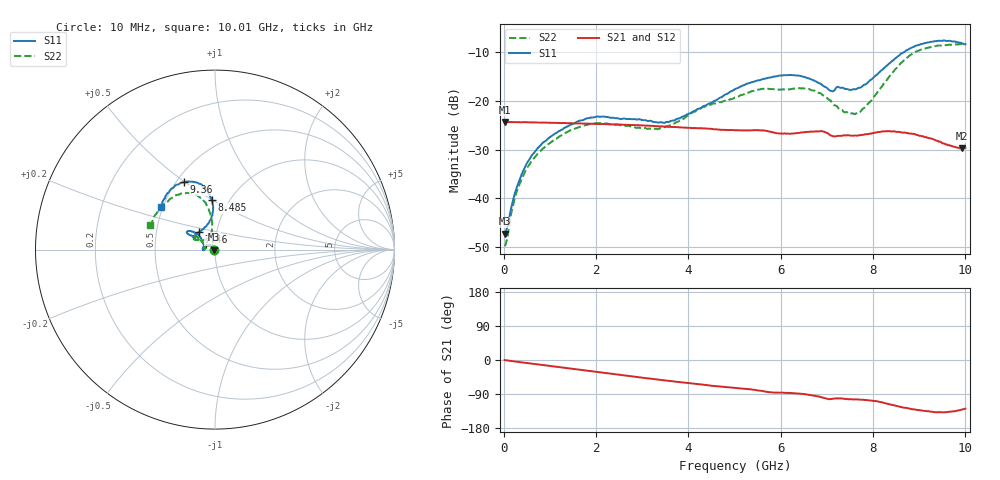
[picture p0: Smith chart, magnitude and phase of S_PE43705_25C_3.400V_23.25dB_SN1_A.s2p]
! Device ID: PE43705
! Serial: 1
! Insertion: A
! Impedance: 50 ohm
! Temp: 25C
! VDD: 3.400V
! Attenuation Step: 23.25dB
#  Hz  S  RI  R  50
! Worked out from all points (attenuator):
!   401 points, 10 MHz to 10.01 GHz, reference 50 ohm
!   highest |S21| = -24.30 dB at 10 MHz (marker M1); lowest = -29.8 dB at 9.935 GHz (marker M2)
!   lowest |S11| = -47.3 dB at 10 MHz (marker M3), VSWR 1.01, Z = 49.6 + j0.0472 ohm
!   |S11| at or under -10 dB: start of sweep to 8.665 GHz
!   |S22| runs from -49.9 to -8.3 dB; largest |S21 - S12| = 0.00087
!   S11 on the Smith chart (normalised r, x): 10 MHz: 0.99, +0.00; 7.46 GHz: 0.82, +0.17; 8.485 GHz: 0.83, +0.49; 9.36 GHz: 0.55, +0.50; 10.01 GHz: 0.49, +0.27
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1e7  -0.00428 0.000476  0.0609 -0.000247  0.061 -0.000191  -0.00317 0.0005
2.6e8  -0.00557 0.0111  0.0604 -0.0046  0.0603 -0.00453  -0.00395 0.0105
5.35e8  -0.0124 0.0211  0.0597 -0.00922  0.0596 -0.00917  -0.00996 0.0193
1.01e9  -0.0331 0.0274  0.0573 -0.0167  0.0573 -0.0167  -0.0281 0.0246
1.685e9  -0.0608 0.0173  0.0524 -0.0263  0.0525 -0.0262  -0.0526 0.017
2.16e9  -0.069 0.00384  0.0481 -0.0323  0.0481 -0.0323  -0.058 0.00725
3.36e9  -0.0598 0.00426  0.0338 -0.0433  0.0339 -0.0432  -0.0501 0.0132
3.835e9  -0.0624 0.0257  0.0279 -0.0457  0.0279 -0.0457  -0.058 0.0275
4.385e9  -0.0729 0.0533  0.021 -0.0476  0.0213 -0.0475  -0.0746 0.0482
5.01e9  -0.0995 0.0876  0.0141 -0.0481  0.0144 -0.048  -0.0885 0.0634
5.535e9  -0.129 0.1006  0.00812 -0.0495  0.0081 -0.0493  -0.1081 0.0741
6.01e9  -0.1519 0.1022  0.00324 -0.0462  0.00336 -0.0459  -0.1105 0.0708
6.685e9  -0.1431 0.0823  -0.0029 -0.0483  -0.00282 -0.0484  -0.1144 0.0584
7.085e9  -0.1096 0.065  -0.0101 -0.0432  -0.00999 -0.0434  -0.0847 0.055
7.46e9  -0.0883 0.0987  -0.0102 -0.0433  -0.00994 -0.043  -0.0504 0.0565
7.785e9  -0.0449 0.1367  -0.0116 -0.0434  -0.0113 -0.043  -0.0284 0.0784
8.36e9  -0.0108 0.2444  -0.0222 -0.0438  -0.0218 -0.0437  -0.0212 0.1781
8.485e9  -0.0166 0.2743  -0.0247 -0.0419  -0.0244 -0.042  -0.0301 0.2095
8.885e9  -0.0689 0.3538  -0.0297 -0.0352  -0.0295 -0.0349  -0.0923 0.297
9.36e9  -0.1713 0.3755  -0.0291 -0.0268  -0.029 -0.0268  -0.2006 0.3073
9.935e9  -0.2938 0.2629  -0.021 -0.0248  -0.0213 -0.0247  -0.3455 0.166
1.001e10  -0.3021 0.2389  -0.0205 -0.0258  -0.0208 -0.0258  -0.3608 0.1369
